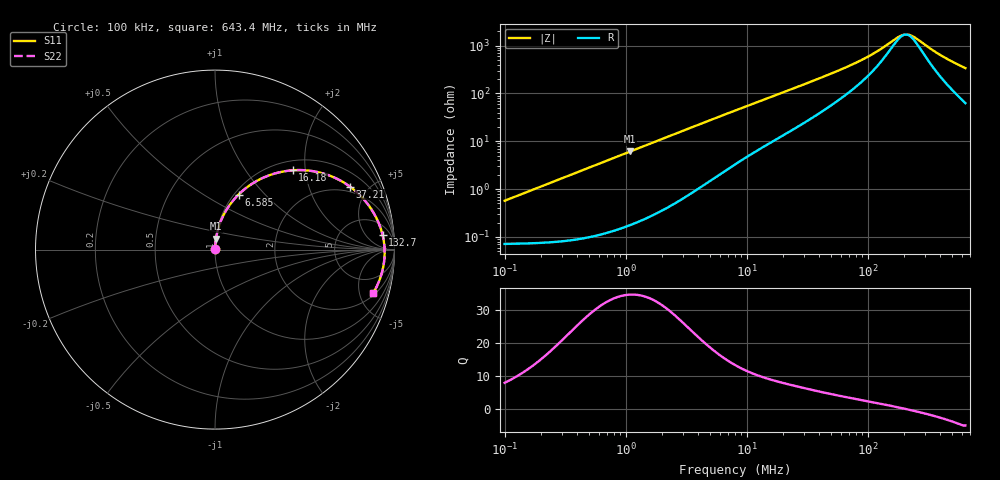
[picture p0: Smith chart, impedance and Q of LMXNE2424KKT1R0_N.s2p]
! LMXNE2424KKT1R0_N  S-PARAMETER MODEL  ( General Type )
! Model Generated by TAIYO YUDEN Corporation (http://www.ty-top.com)
! Version 1.0
! TAIYO YUDEN Control No. 191023NI43SB-FBB
! Copyright(c) 2019 TAIYO YUDEN CO.,LTD. All Rights Reserved.
! Product Description (link to TY-COMPAS)
! https://ds.yuden.co.jp/TYCOMPAS/or/detail?pn=LMXNE2424KKT1R0NN&u=M
! Products Name : Inductors
! Characteristics :
!  Inductance : 1.0 uH , SRF(min) : 106 MHz , DC Resistance(max) : 0.084 Ohm
!  Rated Current : Saturation :1800 mA , Temp Rise : 1410 mA
!  Case Size : 2.4 x 2.4 / 0.094 x 0.094 [mm/inch] , Thickness : 1 / 0.039 [mm/inch]
!  (Conditions: Temperature = 25 degC , DC Bias Current/Voltage = 0A / 0V)
! External Node Assignments :
!  1  o---GGG---o  2
! GND o---------o GND
! Frequency Range : 0.1MHz  -  643.381979MHz  [ 402 STEP ]
# MHz S RI R 50
! Freq[MHz].  S11 Real  S11 Imag  S21 Real  S21 Imag  S12 Real  S12 Imag  S22 Real  S22 Imag
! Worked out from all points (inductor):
!   401 points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, 100 kHz to 643.4 MHz, reference 50 ohm
!   read as one part in series: L = 900 nH near 104.5 kHz
!   highest Q = 34.7 at 1.091 MHz (marker M1), where L = 893 nH
!   self-resonance near 206.4 MHz
!   S11 on the Smith chart (normalised r, x): 100 kHz: 1.00, +0.01; 6.585 MHz: 1.05, +0.72; 16.18 MHz: 1.19, +1.71; 37.21 MHz: 1.69, +3.80; 132.7 MHz: 11, +15; 643.4 MHz: 2.26, -6.67
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0.1  0.000744 0.00565  0.9993 -0.00565  0.9993 -0.00565  0.000744 0.00565
0.434429  0.00152 0.0245  0.9985 -0.0245  0.9985 -0.0245  0.00152 0.0245
1.090957  0.00548 0.0608  0.9945 -0.0608  0.9945 -0.0608  0.00548 0.0608
1.887283  0.0142 0.1037  0.9858 -0.1037  0.9858 -0.1037  0.0142 0.1037
3.890772  0.053 0.2026  0.947 -0.2026  0.947 -0.2026  0.053 0.2026
6.58482  0.1314 0.3068  0.8686 -0.3068  0.8686 -0.3068  0.1314 0.3068
8.02111  0.1791 0.3478  0.8209 -0.3478  0.8209 -0.3478  0.1791 0.3478
11.90188  0.308 0.4161  0.692 -0.4161  0.692 -0.4161  0.308 0.4161
16.17752  0.4325 0.4419  0.5675 -0.4419  0.5675 -0.4419  0.4325 0.4419
22.97475  0.5811 0.4299  0.4189 -0.4299  0.4189 -0.4299  0.5811 0.4299
34.846  0.7325 0.3644  0.2675 -0.3644  0.2675 -0.3644  0.7325 0.3644
37.21487  0.7521 0.3508  0.2479 -0.3508  0.2479 -0.3508  0.7521 0.3508
52.85125  0.8358 0.2724  0.1642 -0.2724  0.1642 -0.2724  0.8358 0.2724
76.72116  0.8919 0.19  0.1081 -0.19  0.1081 -0.19  0.8919 0.19
102.0212  0.9184 0.1316  0.0816 -0.1316  0.0816 -0.1316  0.9184 0.1316
132.7225  0.9338 0.0811  0.0662 -0.0811  0.0662 -0.0811  0.9338 0.0811
151.3811  0.9389 0.0567  0.0611 -0.0567  0.0611 -0.0567  0.9389 0.0567
192.6657  0.9443 0.0126  0.0557 -0.0126  0.0557 -0.0126  0.9443 0.0126
224.6222  0.9452 -0.0155  0.0548 0.0155  0.0548 0.0155  0.9452 -0.0155
250.6447  0.9447 -0.0359  0.0553 0.0359  0.0553 0.0359  0.9447 -0.0359
405.9984  0.9287 -0.1327  0.0713 0.1327  0.0713 0.1327  0.9287 -0.1327
643.382  0.8818 -0.2422  0.1182 0.2422  0.1182 0.2422  0.8818 -0.2422
